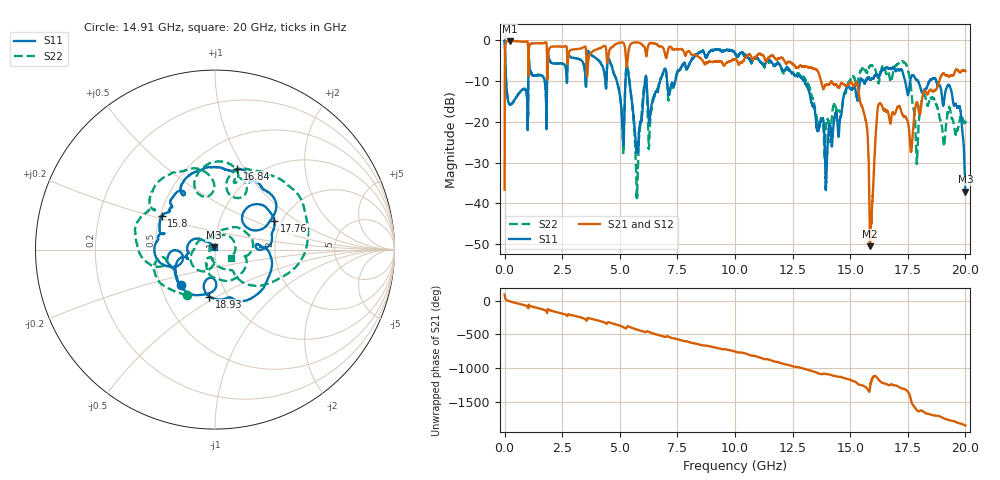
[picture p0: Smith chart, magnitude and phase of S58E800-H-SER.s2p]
!{S58E800}
!Johanson Technology Inc.
!www.johansontechnology.com
!Test Board Conditions:
!Substrate Type  RO4350B
!Substrate Thickness  60 mil
!Substrate Dk  3.66
!TL Type: GCPW
!TL Trace Width  115 mil
!TL Gap  52 mil
!Electrode orientation  Horizontal
!DUT TOPOLOGY	SERIES
!Mounting Pad LxW  55x428 mil
! Created Wed Apr 14 12:03:22 2021
# mhz S ma R 50
! 2 Port Network Data from SP1.SP block
! freq  magS11  angS11  magS21  angS21  magS12  angS12  magS22  angS22
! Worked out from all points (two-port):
!   20001 points, 300 kHz to 20 GHz, reference 50 ohm
!   highest |S21| = -0.12 dB at 226.3 MHz (marker M1); lowest = -50.5 dB at 15.86 GHz (marker M2)
!   |S21| within 3 dB of the highest: 19.94 MHz to 1.029 GHz (1.009 GHz wide, 192 % of centre); 1.898 GHz to 2.712 GHz (813.6 MHz wide, 35.3 % of centre)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
!   lowest |S11| = -37.1 dB at 20 GHz (marker M3), VSWR 1.03, Z = 49.3 + j1.21 ohm
!   |S11| at or under -10 dB: 64.89 MHz to 1.028 GHz (963.4 MHz wide, 176 % of centre); 13.02 GHz to 15.43 GHz (2.413 GHz wide, 17 % of centre); 18.74 GHz to end of sweep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
!   |S22| runs from -38.7 to 0.0 dB; largest |S21 - S12| = 0.012
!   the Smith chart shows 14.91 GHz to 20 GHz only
!   S11 on the Smith chart (normalised r, x): 14.91 GHz: 0.64, -0.27; 15.8 GHz: 0.51, +0.22; 16.84 GHz: 0.81, +0.93; 17.76 GHz: 1.83, +0.67; 18.93 GHz: 0.82, -0.46; 20 GHz: 0.99, +0.02
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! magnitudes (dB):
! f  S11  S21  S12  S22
! 300 kHz  0.0  -36.6  -36.5  0.0
! 226.3 MHz  -15.7  -0.1  -0.1  -15.7
! 3.334 GHz  -4.9  -1.9  -1.9  -4.9
! 4.573 GHz  -5.3  -2.2  -2.1  -5.3
! 5.117 GHz  -21.2  -0.5  -0.5  -21.9
! 5.35 GHz  -7.4  -4.1  -4.1  -6.8
! 5.739 GHz  -27.1  -0.5  -0.5  -37.8
! 6.074 GHz  -11.1  -1.6  -1.6  -10.7
! 6.667 GHz  -12.2  -1.4  -1.4  -11.3
! 10 GHz  -3.1  -4.6  -4.6  -3.1
! 13.33 GHz  -15.5  -6.7  -6.7  -13.8
! 13.97 GHz  -32.6  -10.9  -10.9  -20.2
! 14.91 GHz  -11.2  -10.8  -10.8  -10.5
! 15.8 GHz  -9.1  -28.3  -28.3  -6.8
! 15.86 GHz  -9.6  -50.5  -51.7  -6.2
! 16.24 GHz  -9.1  -15.6  -15.6  -10.5
! 16.67 GHz  -6.8  -18.2  -18.4  -7.8
! 16.84 GHz  -6.6  -17.6  -17.7  -8.5
! 17.76 GHz  -8.7  -19.2  -19.0  -17.1
! 18.93 GHz  -11.6  -9.0  -8.9  -20.1
! 19.74 GHz  -16.2  -7.7  -7.6  -20.0
! 20 GHz  -37.1  -7.6  -7.5  -20.0
